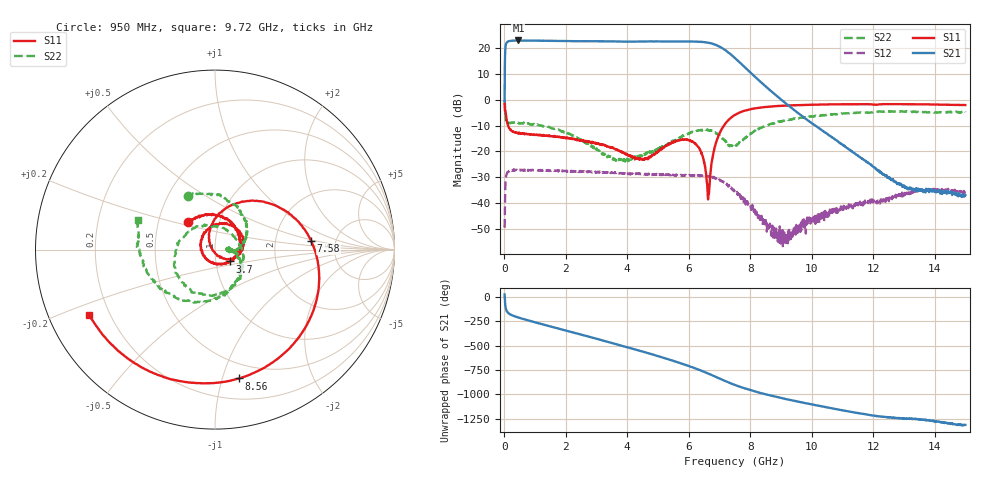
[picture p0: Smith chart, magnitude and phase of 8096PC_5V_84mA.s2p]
!Keysight Technologies,N5247B,US58420632,A.15.75.19
!Date: Wednesday, November 02, 2022 15:35:49
!Correction: S11(C  2-Port  )
!S21(C  2-Port  )
!S12(C  2-Port  )
!S22(C  2-Port  )
!S2P File: Measurements: S11, S21, S12, S22:
# Hz S  dB  R 50
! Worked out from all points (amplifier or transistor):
!   1500 points, 10 MHz to 15 GHz, reference 50 ohm
!   highest |S21| = 22.9 dB at 460 MHz (marker M1)
!   |S21| within 3 dB of that: 35.38 MHz to 7.096 GHz (7.06 GHz wide, 198 % of centre)
!   unconditionally stable (mu >= 1): 10.92 MHz to end of sweep
!   at 2.51 GHz: K = 1.14, MAG = 22.9 dB, |S12| = -27.8 dB
!   at 7.51 GHz: K = 3.54, MAG = 17.4 dB, |S12| = -35.6 dB
!   at 15 GHz: K = 547.22, MAG = -31.0 dB, |S12| = -35.7 dB
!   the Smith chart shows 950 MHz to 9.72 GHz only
!   S11 on the Smith chart (normalised r, x): 950 MHz: 0.71, +0.23; 3.7 GHz: 1.17, -0.16; 7.58 GHz: 3.27, +0.44; 8.56 GHz: 0.37, -1.14; 9.72 GHz: 0.12, -0.24
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1e7  -1.65 -33.3  -0.57 26.2  -49.49 -118.1  -0.08 -38.2
9e7  -8.67 -116.1  22.24 -150.1  -28.24 48.4  -8.99 -139.5
1.5e8  -10.83 -141.3  22.65 -169.5  -27.56 22.7  -8.94 -157.8
4.6e8  -13.05 171.3  22.91 149.2  -27.22 -22.5  -8.87 159.5
9.5e8  -13.45 134.6  22.82 104.8  -27.33 -62.1  -9.47 116.6
1.83e9  -14.53 81.3  22.72 30.0  -27.54 -129.4  -11.94 55.5
2.51e9  -15.77 43.5  22.61 -27.1  -27.76 179.6  -15.87 12.5
3.13e9  -17.43 1.6  22.61 -80.1  -28.06 131.3  -19.96 -6.5
3.7e9  -19.44 -38.4  22.50 -129.6  -28.31 86.0  -23.08 -2.6
4.37e9  -22.92 -117.9  22.50 171.5  -28.51 32.8  -21.99 3.2
5.01e9  -19.79 133.0  22.52 111.4  -28.97 -21.2  -19.07 -8.4
5.52e9  -16.13 71.3  22.51 61.2  -29.20 -66.8  -15.91 -27.4
6.1e9  -16.21 5.0  22.48 -0.8  -29.42 -121.7  -12.55 -71.2
6.75e9  -24.10 120.2  21.71 -82.8  -30.27 170.0  -12.03 -150.0
7.12e9  -10.49 61.8  19.73 -134.9  -31.61 124.1  -15.17 140.0
7.51e9  -5.82 12.8  16.06 174.8  -35.57 84.1  -18.03 37.9
7.58e9  -5.38 5.1  15.29 166.7  -36.70 77.6  -17.59 18.5
8.56e9  -2.73 -79.4  4.57 74.9  -49.31 29.6  -9.90 -114.6
9.72e9  -2.05 -152.4  -6.59 -6.6  -47.71 59.1  -6.78 158.7
1.001e10  -1.96 -168.7  -9.10 -24.8  -45.32 55.9  -6.46 140.1
1.251e10  -1.71 61.9  -30.14 -157.0  -39.23 -72.9  -4.53 -2.5
1.5e10  -2.07 -65.7  -36.94 124.3  -35.74 133.6  -4.83 -141.2
